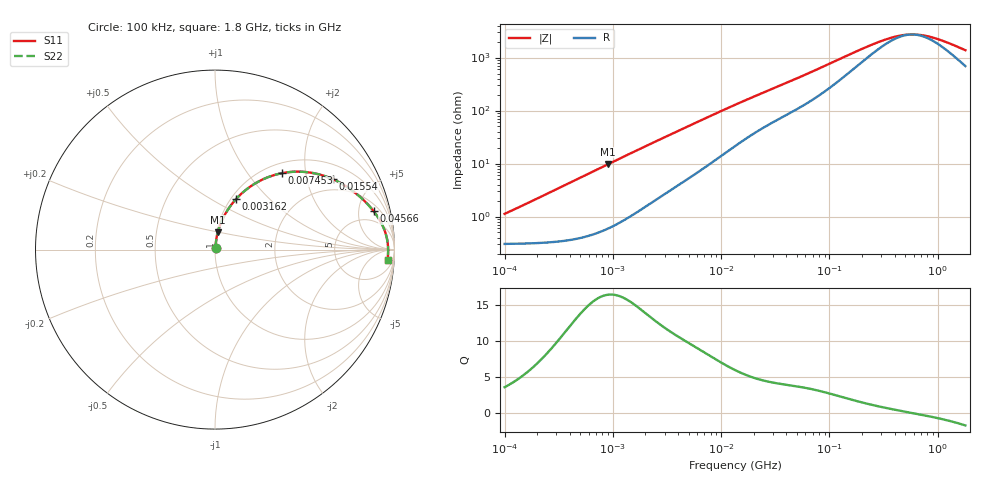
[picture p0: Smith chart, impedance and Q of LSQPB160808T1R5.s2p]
! LSQPB160808T1R5  S-PARAMETER MODEL  ( General Type )
! Model Generated by TAIYO YUDEN Corporation (http://www.ty-top.com)
! Version 4.0
! TAIYO YUDEN Control No. 100810NF18SB-HKC
! Copyright(c) 2007 TAIYO YUDEN CO.,LTD. All Rights Reserved.
! Product Description (link to TY-COMPAS)
! https://ds.yuden.co.jp/TYCOMPAS/or/detail?pn=LSQPB160808T1R5M&u=M
! Products Name : Inductors
! Characteristics :
!  Inductance : 1.5 uH , SRF(min) : 120 MHz , DC Resistance(max) : 0.39 Ohm
!  Rated Current : Saturation :700 mA , Temp Rise : 410 mA (40 degC)
!  Case Size : 1.6 x 0.8 / 0.063 x 0.031 [mm/inch] , Thickness : 0.8 / 0.031 [mm/inch]
!  (Conditions: Temperature = 25 degC , DC Bias Current/Voltage = 0A / 0V)
! External Node Assignments :
!  1  o---GGG---o  2
! GND o---------o GND
! Frequency Range : 0.1MHz  -  1800MHz  [ 402 STEP ]
# MHz S RI R 50
! Freq[MHz].  S11 Real  S11 Imag  S21 Real  S21 Imag  S12 Real  S12 Imag  S22 Real  S22 Imag
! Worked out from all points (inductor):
!   401 points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, 100 kHz to 1.8 GHz, reference 50 ohm
!   read as one part in series: L = 1.72 uH near 105 kHz
!   highest Q = 16.4 at 906.6 kHz (marker M1), where L = 1.71 uH
!   self-resonance near 576 MHz
!   S11 on the Smith chart (normalised r, x): 100 kHz: 1.01, +0.02; 3.162 MHz: 1.06, +0.66; 7.453 MHz: 1.18, +1.48; 15.54 MHz: 1.52, +2.88; 45.66 MHz: 2.91, +7.21; 1.8 GHz: 15, -24
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0.1  0.00314 0.0107  0.9969 -0.0107  0.9969 -0.0107  0.00314 0.0107
0.516129  0.00703 0.0551  0.993 -0.0551  0.993 -0.0551  0.00703 0.0551
0.906643  0.0152 0.0954  0.9848 -0.0954  0.9848 -0.0954  0.0152 0.0954
1.672595  0.0415 0.1683  0.9585 -0.1683  0.9585 -0.1683  0.0415 0.1683
2.66389  0.0895 0.2479  0.9105 -0.2479  0.9105 -0.2479  0.0895 0.2479
3.162158  0.1173 0.2814  0.8827 -0.2814  0.8827 -0.2814  0.1173 0.2814
4.795486  0.2159 0.3638  0.7841 -0.3638  0.7841 -0.3638  0.2159 0.3638
7.452807  0.3712 0.4255  0.6288 -0.4255  0.6288 -0.4255  0.3712 0.4255
9.999495  0.491 0.4333  0.509 -0.4333  0.509 -0.4333  0.491 0.4333
13.41641  0.6052 0.4118  0.3948 -0.4118  0.3948 -0.4118  0.6052 0.4118
15.54051  0.656 0.3927  0.344 -0.3927  0.344 -0.3927  0.656 0.3927
25.36465  0.7874 0.3117  0.2126 -0.3117  0.2126 -0.3117  0.7874 0.3117
45.66099  0.8837 0.2143  0.1163 -0.2143  0.1163 -0.2143  0.8837 0.2143
69.24595  0.9233 0.1544  0.0767 -0.1544  0.0767 -0.1544  0.9233 0.1544
121.6389  0.9503 0.0911  0.0497 -0.0911  0.0497 -0.0911  0.9503 0.0911
224.4022  0.961 0.045  0.039 -0.045  0.039 -0.045  0.961 0.045
357.3983  0.9638 0.0206  0.0362 -0.0206  0.0362 -0.0206  0.9638 0.0206
516.0898  0.9645 0.00459  0.0355 -0.00459  0.0355 -0.00459  0.9645 0.00459
612.6219  0.9647 -0.00258  0.0353 0.00258  0.0353 0.00258  0.9647 -0.00258
727.2099  0.9646 -0.00982  0.0354 0.00982  0.0354 0.00982  0.9646 -0.00982
1050.104  0.9641 -0.0266  0.0359 0.0266  0.0359 0.0266  0.9641 -0.0266
1800  0.9613 -0.0584  0.0387 0.0584  0.0387 0.0584  0.9613 -0.0584
